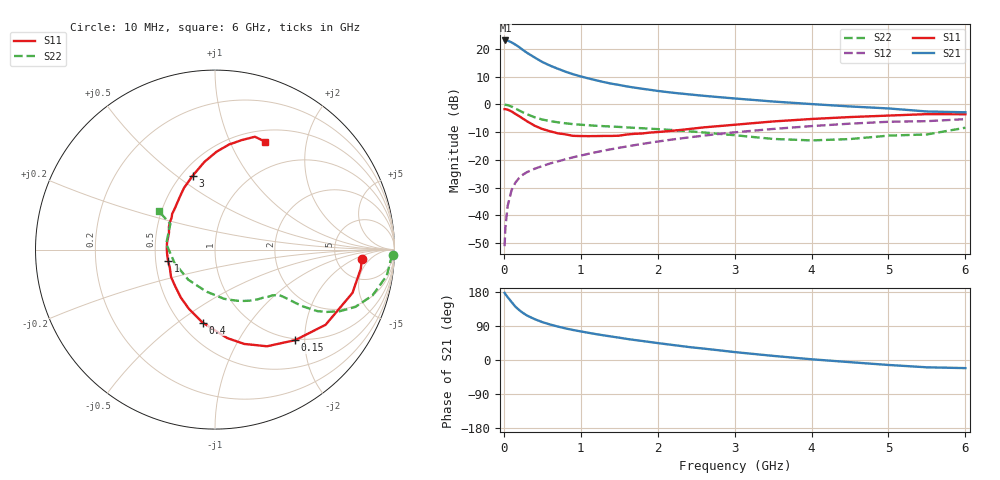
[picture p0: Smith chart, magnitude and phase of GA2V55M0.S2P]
! Infineon Technologies  Discrete & RF Semiconductors
! BF775
! Si NPN RF Bipolar Junction Transistor in SOT23
! VCE = 2.5 V  IC = 5 mA
! Common Emitter S-Parameters:  May  1996
# GHz  S  MA  R  50
!  f  S11  S21  S12  S22
! GHz  MAG  ANG  MAG  ANG  MAG  ANG  MAG  ANG
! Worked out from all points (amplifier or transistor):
!   36 points, 10 MHz to 6 GHz, reference 50 ohm
!   highest |S21| = 23.0 dB at 20 MHz (marker M1)
!   |S21| within 3 dB of that: start of sweep to 228.1 MHz
!   unconditionally stable (mu >= 1): 785.2 MHz to 3.723 GHz
!   at 250 MHz: K = 0.49, MSG = 22.4 dB, |S12| = -25.3 dB
!   at 1.4 GHz: K = 1.14, MAG = 9.5 dB, |S12| = -16.1 dB
!   at 6 GHz: K = 0.98, MSG = 1.2 dB, |S12| = -5.3 dB
!   lowest NFmin = 1.50 dB at 450 MHz
!   S11 on the Smith chart (normalised r, x): 10 MHz: 9.13, -2.94; 150 MHz: 0.97, -1.80; 400 MHz: 0.63, -0.62; 1 GHz: 0.58, -0.08; 3 GHz: 0.57, +0.57; 6 GHz: 0.64, +1.36
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0.01  0.8197 -3.7  14.11 177.2  0.0028 91.1  0.9914 -1.7
0.02  0.8196 -7.4  14.13 174.0  0.0061 85.4  0.981 -3.4
0.05  0.8031 -17.5  14.02 165.8  0.0149 81.5  0.968 -8.6
0.1  0.7451 -34.2  13.05 153.0  0.0284 73.7  0.9141 -16.2
0.15  0.6737 -48.5  11.89 140.8  0.039 66.3  0.845 -22.2
0.2  0.6117 -61.7  10.71 131.7  0.0475 62.1  0.7751 -26.3
0.25  0.5506 -72.7  9.49 124.0  0.0545 58.8  0.7141 -29.1
0.3  0.4978 -82.1  8.5 117.5  0.0601 57.0  0.6658 -31.0
0.4  0.4124 -99.7  6.986 107.9  0.0693 55.2  0.5854 -32.8
0.5  0.3602 -113.9  5.793 100.0  0.0775 54.8  0.5324 -33.6
0.6  0.328 -125.5  4.987 93.8  0.0862 54.7  0.5005 -34.0
0.8  0.2887 -147.9  3.881 83.5  0.1025 55.6  0.4565 -34.8
1  0.2689 -166.4  3.183 75.4  0.1197 56.3  0.4297 -36.1
1.1  0.2679 -174.7  2.93 71.8  0.1288 56.5  0.4203 -37.2
1.3  0.27 171.8  2.519 65.0  0.1472 56.2  0.4048 -39.4
1.6  0.2869 153.4  2.102 55.6  0.1746 55.1  0.3842 -43.9
2.2  0.3351 128.8  1.617 39.5  0.2338 51.3  0.3445 -55.7
3  0.4295 106.9  1.277 20.9  0.3136 43.2  0.2785 -79.6
3.5  0.4922 96.9  1.125 10.9  0.3607 37.1  0.2385 -102.0
4.5  0.5906 82.4  0.917 -5.7  0.4494 24.1  0.2373 -161.5
5.5  0.6671 70.5  0.744 -19.3  0.4984 9.2  0.2873 150.0
6  0.6629 65.1  0.72 -21.4  0.5421 5.2  0.3795 145.7
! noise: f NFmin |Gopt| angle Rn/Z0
0.45  1.5  0.28  29  0.34
0.9  1.8  0.25  59  0.34
